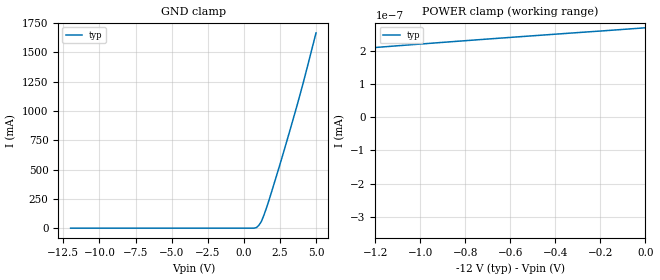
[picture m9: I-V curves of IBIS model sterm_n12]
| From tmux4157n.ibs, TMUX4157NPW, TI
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| sterm_n12
[Model]   sterm_n12
Model_type   Terminator
|   typ   min   max
C_comp   4.826588e-12   NA   NA
[Voltage Range]   -12   NA   NA
[Temperature Range]   27   NA   NA
[Power Clamp Reference]   -12   NA   NA
[GND Clamp Reference]   0   NA   NA
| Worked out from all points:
|   POWER clamp passes 1 mA (typ) near -12.73 V on its own axis
[GND Clamp]
|   Voltage   I(typ)   I(min)   I(max)
-12V      -1.179nA   NA         NA
535.4mV   13.81uA    NA         NA
878.8mV   5.367mA    NA         NA
1.051V    25.46mA    NA         NA
1.222V    58.71mA    NA         NA
1.394V    111.4mA    NA         NA
1.737V    236.5mA    NA         NA
2.253V    442.7mA    NA         NA
2.939V    727mA      NA         NA
3.798V    1.097A     NA         NA
4.313V    1.335A     NA         NA
5V        1.667A     NA         NA
[POWER Clamp]
|   Voltage   I(typ)   I(min)   I(max)
-17V      -1.832A    NA         NA
-7.556V   -348.9pA   NA         NA
-6.697V   -237.9pA   NA         NA
-5.838V   -140.4pA   NA         NA
-4.98V    -55.05pA   NA         NA
-4.121V   19.38pA    NA         NA
-3.263V   84.31pA    NA         NA
-2.232V   151.6pA    NA         NA
-1.202V   209.7pA    NA         NA
0V        269.1pA    NA         NA
